(* Logix 5000 AddOnInstructionDefinition export EH_Picomag_DMA_IOL; software revision 38.00 *)

TYPE EH_CommAOI_Data :
STRUCT
   Device_Comm_Error : BOOL;
   CommSuccess : BOOL;
   CommFailed : BOOL;
   CommTimeOut : BOOL;
   StateDone : BOOL;
   NewState : BOOL;
   OldState : SINT;
   PortSize : SINT;
   DevicePort : SINT;
   MaxState : SINT;
   State : SINT;
   VendorID : INT;
   DeviceID : DINT;
   CyclicData : INT[16];
   AcyclicData : DINT[8];
   ReplayIndex : INT;
   AOI_Diagnostic : DINT;
   ConnectionStatus : DINT;
   OutputData : INT[16];
END_STRUCT
END_TYPE

ADD_ON_INSTRUCTION EH_Picomag_DMA_IOL   (* revision 1.0, vendor Endress+Hauser *)
// Picomag DMA  Rev 1 IO-Link
// Picomag DMA  Rev 2 IO-Link
VAR_IN_OUT
   DataToSend : INT[10]; {required}
   CommAOIBusy : DINT; {required}
   ActiveComPort : DINT; {required}
   DeviceAOISendRequest : DINT; {required}
   CommError : INT; {required}
   DeviceData : EH_CommAOI_Data; {required}
END_VAR
VAR_OUTPUT
   qVendor_ID : DINT; {access Read Only, visible}
   qDevice_ID : DINT; {access Read Only, visible}
END_VAR
VAR_INPUT
   iExecuteRisingEdge : BOOL; {visible}
   iSetSimulation : BOOL; {visible}
   iSetResetTotalizer : BOOL; {visible}
   iSetSimulationConductivity : REAL; {visible}
   iSetSimulationVolumeflow : REAL; {visible}
   iSetSimulationTemperature : REAL; {visible}
END_VAR
VAR_OUTPUT
   qConductivity : REAL; {visible}
   qTotalizer : REAL; {access Read Only, visible}
   qVolumeflow : REAL; {visible}
   qTemperature : REAL; {visible}
   qS_Out_1 : BOOL; {access Read Only, visible}
   qS_Out_2 : BOOL; {visible}
   qSimulationActive : BOOL; {access Read Only, visible}
   qActual_Diagnostics_Code : DINT; {access Read Only, visible}
END_VAR
VAR_IN_OUT
   qActual_Diagnostics_String : STRING; {required}
END_VAR
VAR_OUTPUT
   qLast_Diagnostics_Code : DINT; {visible}
END_VAR
VAR_IN_OUT
   qLast_Diagnostics_String : STRING; {required}
END_VAR
VAR_OUTPUT
   qAOI_Diagnostic : DINT; {access Read Only, visible}
   qCommError : INT; {access None, visible}
   qCommunicationBusy : DINT; {access Read Only, visible}
   qDeviceConnectionError : BOOL; {access Read Only, visible}
END_VAR
VAR
   Calc_DID : DINT; {access None}
   Calc_VID : DINT; {access None}
   Calc_Data : DINT; {access None}
   Calc_VID_1 : DINT; {access None}
   Calc_DID_1 : DINT; {access None}
   Calc_DID_2 : DINT; {access None}
   Cond_DINT : DINT; {access None}
   Temp_DINT : DINT; {access None}
   Calc_Cond : DINT; {access None}
   Cald_Temp : DINT; {access None}
   Calc_Temp : DINT; {access None}
   Calc_CondenStatus : DINT; {access None}
   CMD_Index : INT; {access None}
   CMD_Subindex : INT; {access None}
   CMD_Rd_Wr : BOOL; {access None}
   CMD_ByteLength : INT; {access None}
   StateMax : INT; {access None}
   CMD_RdWr_Buffer : INT[15]; {access None}
   Trigger : BOOL; {access None}
   CMD_Rd : BOOL; {access None}
   CMD_Wr : BOOL; {access None}
   SimulationDINT : DINT; {access None}
   SimulationReal : DINT; {access None}
   Calc_Out : DINT; {access None}
   Calc_Vflow : DINT; {access None}
   Calc_Tota : DINT; {access None}
   Totalizer_DINT : DINT; {access None}
   Vflow_DINT : DINT; {access None}
   xTemp : REAL; {access None}
   InputByteLength : DINT; {access None}
   iState : DINT; {access None}
   AOI_Prio : BOOL; {access None}
   ActiveAOI : BOOL; {access None}
   StateMin : INT; {access None}
   qDevice_ID_select : INT; {access None}
   DeviceID1 : DINT; {access None}
   firstTimeDone : BOOL; {access None}
   Calc_Connection_Status : DINT; {access None}
   ChangedStatus : BOOL; {access None}
   OldStatus : DINT; {access None}
   DeviceID2 : DINT; {access None}
   FALSE : BOOL; {access None}
   TRUE : BOOL := 1; {access None}
END_VAR

ROUTINE Logic   (* structured text *)
// Picomag Communication via AL1323
   // =======================================================================
   // Endress+Hauser Digital Solutions
   // ©Copyright (2024) All Rights Reserved
   // =======================================================================
   // Name:                EH_Picomag_DMA_IOL
   // Version:             1.0
   // Datum:               11.2025
   // Library:             01.01.00
   // Engineering:         Studio5000 V38.00.00
   // Author:              EH
   // =======================================================================
   
   
   qAOI_Diagnostic := DeviceData.AOI_Diagnostic;
   qCommunicationBusy := CommAOIBusy;
   DeviceID1 := 65792;  //0x94FF DevRev 2
   DeviceID2 := 65793;  //0x94FF DevRev 1
   StateMin := 0;
   DeviceData.MaxState := 9;
   
   if DeviceData.DevicePort = 0 or DeviceData.DeviceID < DeviceID1 or DeviceData.DeviceID > DeviceID2 or DeviceData.ConnectionStatus <> 1 then
   
   	qVendor_ID	:= 0;
   	qDevice_ID	:= 0;
   	qConductivity	:= 0;
   	qTotalizer	:= 0;
   	qVolumeflow	:= 0;
   	qTemperature	:= 0;
   	qS_Out_1	:= 0;
   	qS_Out_2	:= 0;
   	qSimulationActive	:= 0;
   	qActual_Diagnostics_Code	:= 0;
   	qLast_Diagnostics_Code	:= 0;
   	qLast_Diagnostics_String	:= '';
   
   	if DeviceData.DevicePort = 0 then
   
   		qActual_Diagnostics_String	:= 'Device Port is Zero';
   		DeviceData.AOI_Diagnostic.1 := TRUE;
   
   	elsif DeviceData.ConnectionStatus <> 1 then
   
   		qActual_Diagnostics_String	:= 'No Device connected';
   		qDeviceConnectionError := TRUE;
   
   	elsif DeviceData.DeviceID < DeviceID1 or DeviceData.DeviceID > DeviceID2  then
   
   		qActual_Diagnostics_String	:= 'Wrong DeviceID';
   		DeviceData.AOI_Diagnostic.2 := TRUE;
   		qVendor_ID := DeviceData.VendorID;
   		qDevice_ID := DeviceData.DeviceID;
   
   	end_if;
   
   else
   
   	if qActual_Diagnostics_Code = 0 then
   
   		qActual_Diagnostics_String	:= '--------';
   
   	end_if;
   
   	if qLast_Diagnostics_Code = 0 then
   
   		qLast_Diagnostics_String	:= '--------';
   
   	end_if;
   
   	DeviceData.AOI_Diagnostic.1 := FALSE;
   	qDeviceConnectionError := FALSE;
   	DeviceData.AOI_Diagnostic.2  := FALSE;
   
   end_if;
   
   
   if not DeviceData.AOI_Diagnostic.0
   	and not qDeviceConnectionError
   	and not DeviceData.AOI_Diagnostic.2
   	and DeviceData.DevicePort > 0 or ActiveAOI and qDeviceConnectionError then
   
   	//*********************************
   	//Vendor ID
   	//*********************************
   
   	qVendor_ID := DeviceData.VendorID;
   
   	//*********************************
   	//Device ID
   	//*********************************
   	if DeviceData.DeviceID = DeviceID1 then
   
   		qDevice_ID_select := 1;
   
   	elsif DeviceData.DeviceID = DeviceID2 then
   
   		qDevice_ID_select := 2;
   
   	else
   
   		qDevice_ID_select := 0;
   
   	end_if;
   
   	qDevice_ID := DeviceData.DeviceID;
   
   	case qDevice_ID_select of
   
   		//*********************************
   		1: // Picomag Rev 1
   		//*********************************
   
   			Calc_Tota 	:= 0+((DeviceData.DevicePort-1)*InputByteLength);  // Value  95 + Protnumber x Datalength in Byte
   			Calc_Vflow 	:= 2+((DeviceData.DevicePort-1)*InputByteLength);  // Value  97 + Protnumber x Datalength in Byte
   			Calc_Temp 	:= 4+((DeviceData.DevicePort-1)*InputByteLength);  // Value  99 + Protnumber x Datalength in Byte
   			Calc_Out 	:= 4+((DeviceData.DevicePort-1)*InputByteLength); // Value  99 + Protnumber x Datalength in Byte
   			// Temp und Out are in the Same 2 byte
   
   			//*********************************
   			//Process Data Totalizer
   			//*********************************
   
   			Totalizer_DINT		:= DeviceData.CyclicData[Calc_Tota+1];
   			Totalizer_DINT.8	:= DeviceData.CyclicData[Calc_Tota+1].8;
   			Totalizer_DINT.9 	:= DeviceData.CyclicData[Calc_Tota+1].9;
   			Totalizer_DINT.10	:= DeviceData.CyclicData[Calc_Tota+1].10;
   			Totalizer_DINT.11	:= DeviceData.CyclicData[Calc_Tota+1].11;
   			Totalizer_DINT.12 	:= DeviceData.CyclicData[Calc_Tota+1].12;
   			Totalizer_DINT.13	:= DeviceData.CyclicData[Calc_Tota+1].13;
   			Totalizer_DINT.14	:= DeviceData.CyclicData[Calc_Tota+1].14;
   			Totalizer_DINT.15	:= DeviceData.CyclicData[Calc_Tota+1].15;
   			Totalizer_DINT.16	:= DeviceData.CyclicData[Calc_Tota].0;
   			Totalizer_DINT.17	:= DeviceData.CyclicData[Calc_Tota].1;
   			Totalizer_DINT.18	:= DeviceData.CyclicData[Calc_Tota].2;
   			Totalizer_DINT.19	:= DeviceData.CyclicData[Calc_Tota].3;
   			Totalizer_DINT.20	:= DeviceData.CyclicData[Calc_Tota].4;
   			Totalizer_DINT.21	:= DeviceData.CyclicData[Calc_Tota].5;
   			Totalizer_DINT.22	:= DeviceData.CyclicData[Calc_Tota].6;
   			Totalizer_DINT.23	:= DeviceData.CyclicData[Calc_Tota].7;
   			Totalizer_DINT.24	:= DeviceData.CyclicData[Calc_Tota].8;
   			Totalizer_DINT.25	:= DeviceData.CyclicData[Calc_Tota].9;
   			Totalizer_DINT.26	:= DeviceData.CyclicData[Calc_Tota].10;
   			Totalizer_DINT.27	:= DeviceData.CyclicData[Calc_Tota].11;
   			Totalizer_DINT.28	:= DeviceData.CyclicData[Calc_Tota].12;
   			Totalizer_DINT.29	:= DeviceData.CyclicData[Calc_Tota].13;
   			Totalizer_DINT.30	:= DeviceData.CyclicData[Calc_Tota].14;
   			Totalizer_DINT.31	:= DeviceData.CyclicData[Calc_Tota].15;
   
   			COP(Totalizer_DINT,qTotalizer,1);
   
   			//*********************************
   			//Process Data Volumeflow
   			//*********************************
   
   			Vflow_DINT		:= DeviceData.CyclicData[Calc_Vflow+1];
   			Vflow_DINT.8	:= DeviceData.CyclicData[Calc_Vflow+1].8;
   			Vflow_DINT.9	:= DeviceData.CyclicData[Calc_Vflow+1].9;
   			Vflow_DINT.10	:= DeviceData.CyclicData[Calc_Vflow+1].10;
   			Vflow_DINT.11	:= DeviceData.CyclicData[Calc_Vflow+1].11;
   			Vflow_DINT.12	:= DeviceData.CyclicData[Calc_Vflow+1].12;
   			Vflow_DINT.13	:= DeviceData.CyclicData[Calc_Vflow+1].13;
   			Vflow_DINT.14	:= DeviceData.CyclicData[Calc_Vflow+1].14;
   			Vflow_DINT.15	:= DeviceData.CyclicData[Calc_Vflow+1].15;
   			Vflow_DINT.16	:= DeviceData.CyclicData[Calc_Vflow].0;
   			Vflow_DINT.17	:= DeviceData.CyclicData[Calc_Vflow].1;
   			Vflow_DINT.18	:= DeviceData.CyclicData[Calc_Vflow].2;
   			Vflow_DINT.19	:= DeviceData.CyclicData[Calc_Vflow].3;
   			Vflow_DINT.20	:= DeviceData.CyclicData[Calc_Vflow].4;
   			Vflow_DINT.21	:= DeviceData.CyclicData[Calc_Vflow].5;
   			Vflow_DINT.22	:= DeviceData.CyclicData[Calc_Vflow].6;
   			Vflow_DINT.23	:= DeviceData.CyclicData[Calc_Vflow].7;
   			Vflow_DINT.24	:= DeviceData.CyclicData[Calc_Vflow].8;
   			Vflow_DINT.25	:= DeviceData.CyclicData[Calc_Vflow].9;
   			Vflow_DINT.26	:= DeviceData.CyclicData[Calc_Vflow].10;
   			Vflow_DINT.27	:= DeviceData.CyclicData[Calc_Vflow].11;
   			Vflow_DINT.28	:= DeviceData.CyclicData[Calc_Vflow].12;
   			Vflow_DINT.29	:= DeviceData.CyclicData[Calc_Vflow].13;
   			Vflow_DINT.30	:= DeviceData.CyclicData[Calc_Vflow].14;
   			Vflow_DINT.31	:= DeviceData.CyclicData[Calc_Vflow].15;
   
   			COP(Vflow_DINT,qVolumeflow,1);
   
   			//*********************************
   			// Process Parameter Temperatur
   			//*********************************
   
   			Temp_DINT.0	:= DeviceData.CyclicData[Calc_Temp].4;
   			Temp_DINT.1	:= DeviceData.CyclicData[Calc_Temp].5;
   			Temp_DINT.2	:= DeviceData.CyclicData[Calc_Temp].6;
   			Temp_DINT.3	:= DeviceData.CyclicData[Calc_Temp].7;
   			Temp_DINT.4	:= DeviceData.CyclicData[Calc_Temp].8;
   			Temp_DINT.5	:= DeviceData.CyclicData[Calc_Temp].9;
   			Temp_DINT.6	:= DeviceData.CyclicData[Calc_Temp].10;
   			Temp_DINT.7	:= DeviceData.CyclicData[Calc_Temp].11;
   			Temp_DINT.8	:= DeviceData.CyclicData[Calc_Temp].12;
   			Temp_DINT.9	:= DeviceData.CyclicData[Calc_Temp].13;
   			Temp_DINT.10:= DeviceData.CyclicData[Calc_Temp].14;
   			Temp_DINT.11:= DeviceData.CyclicData[Calc_Temp].15;
   			Temp_DINT.12:= DeviceData.CyclicData[Calc_Temp].15;
   			Temp_DINT.13:= DeviceData.CyclicData[Calc_Temp].15;
   			Temp_DINT.14:= DeviceData.CyclicData[Calc_Temp].15;
   			Temp_DINT.15:= DeviceData.CyclicData[Calc_Temp].15;
   			Temp_DINT.16:= DeviceData.CyclicData[Calc_Temp].15;
   			Temp_DINT.17:= DeviceData.CyclicData[Calc_Temp].15;
   			Temp_DINT.18:= DeviceData.CyclicData[Calc_Temp].15;
   			Temp_DINT.19:= DeviceData.CyclicData[Calc_Temp].15;
   			Temp_DINT.20:= DeviceData.CyclicData[Calc_Temp].15;
   			Temp_DINT.21:= DeviceData.CyclicData[Calc_Temp].15;
   			Temp_DINT.22:= DeviceData.CyclicData[Calc_Temp].15;
   			Temp_DINT.23:= DeviceData.CyclicData[Calc_Temp].15;
   			Temp_DINT.24:= DeviceData.CyclicData[Calc_Temp].15;
   			Temp_DINT.25:= DeviceData.CyclicData[Calc_Temp].15;
   			Temp_DINT.26:= DeviceData.CyclicData[Calc_Temp].15;
   			Temp_DINT.27:= DeviceData.CyclicData[Calc_Temp].15;
   			Temp_DINT.28:= DeviceData.CyclicData[Calc_Temp].15;
   			Temp_DINT.29:= DeviceData.CyclicData[Calc_Temp].15;
   			Temp_DINT.30:= DeviceData.CyclicData[Calc_Temp].15;
   			Temp_DINT.31:= DeviceData.CyclicData[Calc_Temp].15;
   
   			xTemp	:= Temp_DINT;
   			qTemperature := xTemp/10;
   
   			//*********************************
   			// Process Parameter State IO1 and IO2
   			//*********************************
   
   			qS_Out_1 := DeviceData.CyclicData[Calc_Out].2;
   			qS_Out_2 := DeviceData.CyclicData[Calc_Out].3;
   
   
   
   		//*********************************
   	    2: // Picomag Rev 2
   	    //*********************************
   
   			Calc_Cond 	:= 0+((DeviceData.DevicePort-1)*InputByteLength);  // Value  (95) 0 + Protnumber x Datalength in Byte
   			Calc_Tota 	:= 2+((DeviceData.DevicePort-1)*InputByteLength);  // Value  (97) 2 + Protnumber x Datalength in Byte
   			Calc_Vflow 	:= 4+((DeviceData.DevicePort-1)*InputByteLength);  // Value  (99) 4 + Protnumber x Datalength in Byte
   			Calc_Temp 	:= 6+((DeviceData.DevicePort-1)*InputByteLength); // Value  (101) 6 + Protnumber x Datalength in Byte
   			Calc_Out 	:= 7+((DeviceData.DevicePort-1)*InputByteLength); // Value  (102) 7 + Protnumber x Datalength in Byte
   
   
   			//*********************************
   			//Process Data Conductivity
   			//*********************************
   
   			Cond_DINT	:= DeviceData.CyclicData[Calc_Cond+1];
   			Cond_DINT.8	:= DeviceData.CyclicData[Calc_Cond+1].8;
   			Cond_DINT.9	:= DeviceData.CyclicData[Calc_Cond+1].9;
   			Cond_DINT.10 := DeviceData.CyclicData[Calc_Cond+1].10;
   			Cond_DINT.11 := DeviceData.CyclicData[Calc_Cond+1].11;
   			Cond_DINT.12 := DeviceData.CyclicData[Calc_Cond+1].12;
   			Cond_DINT.13 := DeviceData.CyclicData[Calc_Cond+1].13;
   			Cond_DINT.14 := DeviceData.CyclicData[Calc_Cond+1].14;
   			Cond_DINT.15 := DeviceData.CyclicData[Calc_Cond+1].15;
   			Cond_DINT.16 := DeviceData.CyclicData[Calc_Cond].0;
   			Cond_DINT.17 := DeviceData.CyclicData[Calc_Cond].1;
   			Cond_DINT.18 := DeviceData.CyclicData[Calc_Cond].2;
   			Cond_DINT.19 := DeviceData.CyclicData[Calc_Cond].3;
   			Cond_DINT.20 := DeviceData.CyclicData[Calc_Cond].4;
   			Cond_DINT.21 := DeviceData.CyclicData[Calc_Cond].5;
   			Cond_DINT.22 := DeviceData.CyclicData[Calc_Cond].6;
   			Cond_DINT.23 := DeviceData.CyclicData[Calc_Cond].7;
   			Cond_DINT.24 := DeviceData.CyclicData[Calc_Cond].8;
   			Cond_DINT.25 := DeviceData.CyclicData[Calc_Cond].9;
   			Cond_DINT.26 := DeviceData.CyclicData[Calc_Cond].10;
   			Cond_DINT.27 := DeviceData.CyclicData[Calc_Cond].11;
   			Cond_DINT.28 := DeviceData.CyclicData[Calc_Cond].12;
   			Cond_DINT.29 := DeviceData.CyclicData[Calc_Cond].13;
   			Cond_DINT.30 := DeviceData.CyclicData[Calc_Cond].14;
   			Cond_DINT.31 := DeviceData.CyclicData[Calc_Cond].15;
   
   			COP(Cond_DINT,qConductivity,1);
   
   			//*********************************
   			//Process Data Totalizer
   			//*********************************
   
   			Totalizer_DINT := DeviceData.CyclicData[Calc_Tota+1];
   			Totalizer_DINT.8 := DeviceData.CyclicData[Calc_Tota+1].8;
   			Totalizer_DINT.9 := DeviceData.CyclicData[Calc_Tota+1].9;
   			Totalizer_DINT.10 := DeviceData.CyclicData[Calc_Tota+1].10;
   			Totalizer_DINT.11 := DeviceData.CyclicData[Calc_Tota+1].11;
   			Totalizer_DINT.12 := DeviceData.CyclicData[Calc_Tota+1].12;
   			Totalizer_DINT.13 := DeviceData.CyclicData[Calc_Tota+1].13;
   			Totalizer_DINT.14 := DeviceData.CyclicData[Calc_Tota+1].14;
   			Totalizer_DINT.15 := DeviceData.CyclicData[Calc_Tota+1].15;
   			Totalizer_DINT.16 := DeviceData.CyclicData[Calc_Tota].0;
   			Totalizer_DINT.17 := DeviceData.CyclicData[Calc_Tota].1;
   			Totalizer_DINT.18 := DeviceData.CyclicData[Calc_Tota].2;
   			Totalizer_DINT.19 := DeviceData.CyclicData[Calc_Tota].3;
   			Totalizer_DINT.20 := DeviceData.CyclicData[Calc_Tota].4;
   			Totalizer_DINT.21 := DeviceData.CyclicData[Calc_Tota].5;
   			Totalizer_DINT.22 := DeviceData.CyclicData[Calc_Tota].6;
   			Totalizer_DINT.23 := DeviceData.CyclicData[Calc_Tota].7;
   			Totalizer_DINT.24 := DeviceData.CyclicData[Calc_Tota].8;
   			Totalizer_DINT.25 := DeviceData.CyclicData[Calc_Tota].9;
   			Totalizer_DINT.26 := DeviceData.CyclicData[Calc_Tota].10;
   			Totalizer_DINT.27 := DeviceData.CyclicData[Calc_Tota].11;
   			Totalizer_DINT.28 := DeviceData.CyclicData[Calc_Tota].12;
   			Totalizer_DINT.29 := DeviceData.CyclicData[Calc_Tota].13;
   			Totalizer_DINT.30 := DeviceData.CyclicData[Calc_Tota].14;
   			Totalizer_DINT.31 := DeviceData.CyclicData[Calc_Tota].15;
   
   			COP(Totalizer_DINT,qTotalizer,1);
   
   			//*********************************
   			//Process Data Volumeflow
   			//*********************************
   
   			Vflow_DINT	:= DeviceData.CyclicData[Calc_Vflow+1];
   			Vflow_DINT.8 := DeviceData.CyclicData[Calc_Vflow+1].8;
   			Vflow_DINT.9 := DeviceData.CyclicData[Calc_Vflow+1].9;
   			Vflow_DINT.10 := DeviceData.CyclicData[Calc_Vflow+1].10;
   			Vflow_DINT.11 := DeviceData.CyclicData[Calc_Vflow+1].11;
   			Vflow_DINT.12 := DeviceData.CyclicData[Calc_Vflow+1].12;
   			Vflow_DINT.13 := DeviceData.CyclicData[Calc_Vflow+1].13;
   			Vflow_DINT.14 := DeviceData.CyclicData[Calc_Vflow+1].14;
   			Vflow_DINT.15 := DeviceData.CyclicData[Calc_Vflow+1].15;
   			Vflow_DINT.16 := DeviceData.CyclicData[Calc_Vflow].0;
   			Vflow_DINT.17 := DeviceData.CyclicData[Calc_Vflow].1;
   			Vflow_DINT.18 := DeviceData.CyclicData[Calc_Vflow].2;
   			Vflow_DINT.19 := DeviceData.CyclicData[Calc_Vflow].3;
   			Vflow_DINT.20 := DeviceData.CyclicData[Calc_Vflow].4;
   			Vflow_DINT.21 := DeviceData.CyclicData[Calc_Vflow].5;
   			Vflow_DINT.22 := DeviceData.CyclicData[Calc_Vflow].6;
   			Vflow_DINT.23 := DeviceData.CyclicData[Calc_Vflow].7;
   			Vflow_DINT.24 := DeviceData.CyclicData[Calc_Vflow].8;
   			Vflow_DINT.25 := DeviceData.CyclicData[Calc_Vflow].9;
   			Vflow_DINT.26 := DeviceData.CyclicData[Calc_Vflow].10;
   			Vflow_DINT.27 := DeviceData.CyclicData[Calc_Vflow].11;
   			Vflow_DINT.28 := DeviceData.CyclicData[Calc_Vflow].12;
   			Vflow_DINT.29 := DeviceData.CyclicData[Calc_Vflow].13;
   			Vflow_DINT.30 := DeviceData.CyclicData[Calc_Vflow].14;
   			Vflow_DINT.31 := DeviceData.CyclicData[Calc_Vflow].15;
   
   			COP(Vflow_DINT,qVolumeflow,1);
   
   			//*********************************
   			// Process Parameter Temperatur
   			//*********************************
   
   			Temp_DINT	:= DeviceData.CyclicData[Calc_Temp];
   			xTemp		:= Temp_DINT;
   			qTemperature:= xTemp/10;
   
   
   			//*********************************
   			// Process Parameter State IO1 and IO2
   			//*********************************
   
   			qS_Out_1 := DeviceData.CyclicData[Calc_Out].10;
   			qS_Out_2 := DeviceData.CyclicData[Calc_Out].11;
   
   		end_case;
   
   
   	//*********************************
   	// Checking for CommBlockBusy
   	//*********************************
   
   
   	if iExecuteRisingEdge and DeviceData.State = 0 then
   
   		DeviceAOISendRequest.[DeviceData.DevicePort] := 1;
   
   	end_if;
   
   
   	if ActiveComPort = DeviceData.DevicePort then
   
   		AOI_Prio :=1;
   	else
   
   		AOI_Prio := 0;
   	end_if;
   
   
   	if CommAOIBusy = 1 and iExecuteRisingEdge and DeviceData.State = 0 and AOI_Prio then
   
   		ActiveAOI := 1;
   
   
   	end_if;
   
   
   	qCommunicationBusy := CommAOIBusy;
   	qAOI_Diagnostic := DeviceData.AOI_Diagnostic;
   
   	if  ActiveAOI and qDeviceConnectionError then
   
   		DeviceData.State := DeviceData.MaxState;
   
   	end_if;
   
   	//*********************************
   	// State machine
   	//*********************************
   
   	if ActiveAOI or DeviceData.State = DeviceData.MaxState then
   
   	case DeviceData.State of
   
   		//*********************************
   	    0: // Idle
   	    //*********************************
   
   		    // Initializing reset to O for CMD Relevant Settings
   		    Trigger := 0;
   			CMD_Index := 0;
   			CMD_Subindex := 0;
   			CMD_Wr := 0;
   			CMD_Rd := 0;
   		    CMD_ByteLength := 0;
   
   			IF DeviceData.DevicePort = ActiveComPort then // check if Device is Active to reset success
   					DeviceData.CommSuccess := 0;
   					DeviceData.CommTimeOut := 0;
   					DeviceData.NewState := 1;
   					DeviceData.StateDone := 0;
   			end_if;
   
   		    // Wait for trigger
   		    if iExecuteRisingEdge and ActiveComPort = DeviceData.DevicePort then
   
   				DeviceData.AOI_Diagnostic := 0;
   				DeviceData.State := DeviceData.State + 1;
   
   		    end_if;
   
   	    //*********************************
   	    1: // Simulation
   	    //*********************************
   
   		    CMD_Index := 351;
   		    CMD_Subindex := 0;
   		    CMD_Wr := 1;
   			CMD_Rd := 0;
   		    CMD_ByteLength := 2;
   			DataToSend[6]:= 0;
   			DataToSend[7]:= 0;
   
   		    if iSetSimulation then
   
   			   DataToSend[6].8 := 1;
   
   			else
   
   			    DataToSend[6].8 := 0;
   
   			end_if;
   
   		    Trigger := 1;
   
   			if DeviceData.NewState then
   
   				DeviceData.StateDone := 1;
   
   			end_if;
   
   			if  DeviceData.CommSuccess and DeviceData.ReplayIndex = CMD_Index then
   
   				Trigger := 0;
   		        DeviceData.State := DeviceData.State + 1;
   				DeviceData.CommSuccess := 0;
   				DeviceData.AcyclicData[0] := 0;
   				DeviceData.NewState := 1;
   
   			 elsif DeviceData.CommTimeOut then
   
   				DeviceData.AOI_Diagnostic.[DeviceData.State+7] := 1;
   				Trigger := 0;
   		        DeviceData.State := DeviceData.State + 1;
   				DeviceData.CommTimeOut := 0;
   				DeviceData.AcyclicData[0] := 0;
   				DeviceData.NewState := 1;
   
   		    end_if;
   
   	    //*********************************
   	    2: // Simulation - Value VolumeFlow
   	    //*********************************
   
   		    CMD_Index := 358;
   		    CMD_Subindex := 0;
   		    CMD_Wr := 1;
   			CMD_Rd := 0;
   		    CMD_ByteLength := 4;
   
   			COP(iSetSimulationVolumeflow,SimulationDINT,1); // Copy the Bits of the REAL in a DINT not the Value
   
   			DataToSend[6].0 :=  SimulationDINT.24;
   			DataToSend[6].1 :=  SimulationDINT.25;
   			DataToSend[6].2 :=  SimulationDINT.26;
   			DataToSend[6].3 :=  SimulationDINT.27;
   			DataToSend[6].4 :=  SimulationDINT.28;
   			DataToSend[6].5 :=  SimulationDINT.29;
   			DataToSend[6].6 :=  SimulationDINT.30;
   			DataToSend[6].7 :=  SimulationDINT.31;
   			DataToSend[6].8 :=  SimulationDINT.16;
   			DataToSend[6].9 :=  SimulationDINT.17;
   			DataToSend[6].10 := SimulationDINT.18;
   			DataToSend[6].11 := SimulationDINT.19;
   			DataToSend[6].12 := SimulationDINT.20;
   			DataToSend[6].13 := SimulationDINT.21;
   			DataToSend[6].14 := SimulationDINT.22;
   			DataToSend[6].15 := SimulationDINT.23;
   			DataToSend[7].0  := SimulationDINT.8;
   			DataToSend[7].1  := SimulationDINT.9;
   			DataToSend[7].2  := SimulationDINT.10;
   			DataToSend[7].3  := SimulationDINT.11;
   			DataToSend[7].4  := SimulationDINT.12;
   			DataToSend[7].5  := SimulationDINT.13;
   			DataToSend[7].6  := SimulationDINT.14;
   			DataToSend[7].7  := SimulationDINT.15;
   			DataToSend[7].8  := SimulationDINT.0;
   			DataToSend[7].9  := SimulationDINT.1;
   			DataToSend[7].10 := SimulationDINT.2;
   			DataToSend[7].11 := SimulationDINT.3;
   			DataToSend[7].12 := SimulationDINT.4;
   			DataToSend[7].13 := SimulationDINT.5;
   			DataToSend[7].14 := SimulationDINT.6;
   			DataToSend[7].15 := SimulationDINT.7;
   
   		    Trigger := 1;
   
   			if DeviceData.NewState then
   
   				DeviceData.StateDone := 1;
   
   			end_if;
   
   			if  DeviceData.CommSuccess and DeviceData.ReplayIndex = CMD_Index then
   
   				Trigger := 0;
   		        DeviceData.State := DeviceData.State + 1;
   				DeviceData.CommSuccess := 0;
   				DeviceData.AcyclicData[0] := 0;
   				DeviceData.NewState := 1;
   
   			elsif DeviceData.CommTimeOut then
   
   				DeviceData.AOI_Diagnostic.[DeviceData.State+7] := 1;
   				Trigger := 0;
   		        DeviceData.State := DeviceData.State + 1;
   				DeviceData.CommTimeOut := 0;
   				DeviceData.AcyclicData[0] := 0;
   				DeviceData.NewState := 1;
   
   		    end_if;
   
   
   		//*********************************
   	    3: // Simulation - Value Temperature
   	    //*********************************
   
   		    CMD_Index := 360;
   		    CMD_Subindex := 0;
   		    CMD_Wr := 1;
   			CMD_Rd := 0;
   		    CMD_ByteLength := 4;
   
   			COP(iSetSimulationTemperature,SimulationDINT,1); // Copy the Bits of the REAL in a DINT not the Value
   
   			DataToSend[6].0 :=  SimulationDINT.24;
   			DataToSend[6].1 :=  SimulationDINT.25;
   			DataToSend[6].2 :=  SimulationDINT.26;
   			DataToSend[6].3 :=  SimulationDINT.27;
   			DataToSend[6].4 :=  SimulationDINT.28;
   			DataToSend[6].5 :=  SimulationDINT.29;
   			DataToSend[6].6 :=  SimulationDINT.30;
   			DataToSend[6].7 :=  SimulationDINT.31;
   			DataToSend[6].8 :=  SimulationDINT.16;
   			DataToSend[6].9 :=  SimulationDINT.17;
   			DataToSend[6].10 := SimulationDINT.18;
   			DataToSend[6].11 := SimulationDINT.19;
   			DataToSend[6].12 := SimulationDINT.20;
   			DataToSend[6].13 := SimulationDINT.21;
   			DataToSend[6].14 := SimulationDINT.22;
   			DataToSend[6].15 := SimulationDINT.23;
   			DataToSend[7].0  := SimulationDINT.8;
   			DataToSend[7].1  := SimulationDINT.9;
   			DataToSend[7].2  := SimulationDINT.10;
   			DataToSend[7].3  := SimulationDINT.11;
   			DataToSend[7].4  := SimulationDINT.12;
   			DataToSend[7].5  := SimulationDINT.13;
   			DataToSend[7].6  := SimulationDINT.14;
   			DataToSend[7].7  := SimulationDINT.15;
   			DataToSend[7].8  := SimulationDINT.0;
   			DataToSend[7].9  := SimulationDINT.1;
   			DataToSend[7].10 := SimulationDINT.2;
   			DataToSend[7].11 := SimulationDINT.3;
   			DataToSend[7].12 := SimulationDINT.4;
   			DataToSend[7].13 := SimulationDINT.5;
   			DataToSend[7].14 := SimulationDINT.6;
   			DataToSend[7].15 := SimulationDINT.7;
   
   		    Trigger := 1;
   
   			if DeviceData.NewState then
   
   				DeviceData.StateDone := 1;
   
   			end_if;
   
   			if  DeviceData.CommSuccess and DeviceData.ReplayIndex = CMD_Index then
   
   				Trigger := 0;
   		        DeviceData.State := DeviceData.State + 1;
   				DeviceData.CommSuccess := 0;
   				DeviceData.AcyclicData[0] := 0;
   				DeviceData.NewState := 1;
   
   			elsif DeviceData.CommTimeOut then
   
   				DeviceData.AOI_Diagnostic.[DeviceData.State+7] := 1;
   				Trigger := 0;
   		        DeviceData.State := DeviceData.State + 1;
   				DeviceData.CommTimeOut := 0;
   				DeviceData.AcyclicData[0] := 0;
   				DeviceData.NewState := 1;
   
   		    end_if;
   
   		//*********************************
   	    4: // Simulation - Value Conductivity
   	    //*********************************
   
   		    CMD_Index := 359;
   		    CMD_Subindex := 0;
   		    CMD_Wr := 1;
   			CMD_Rd := 0;
   		    CMD_ByteLength := 4;
   
   			COP(iSetSimulationConductivity,SimulationDINT,1); // Copie the Bits from the Real in a DINT
   
   			DataToSend[6].0 :=  SimulationDINT.24;
   			DataToSend[6].1 :=  SimulationDINT.25;
   			DataToSend[6].2 :=  SimulationDINT.26;
   			DataToSend[6].3 :=  SimulationDINT.27;
   			DataToSend[6].4 :=  SimulationDINT.28;
   			DataToSend[6].5 :=  SimulationDINT.29;
   			DataToSend[6].6 :=  SimulationDINT.30;
   			DataToSend[6].7 :=  SimulationDINT.31;
   			DataToSend[6].8 :=  SimulationDINT.16;
   			DataToSend[6].9 :=  SimulationDINT.17;
   			DataToSend[6].10 := SimulationDINT.18;
   			DataToSend[6].11 := SimulationDINT.19;
   			DataToSend[6].12 := SimulationDINT.20;
   			DataToSend[6].13 := SimulationDINT.21;
   			DataToSend[6].14 := SimulationDINT.22;
   			DataToSend[6].15 := SimulationDINT.23;
   			DataToSend[7].0  := SimulationDINT.8;
   			DataToSend[7].1  := SimulationDINT.9;
   			DataToSend[7].2  := SimulationDINT.10;
   			DataToSend[7].3  := SimulationDINT.11;
   			DataToSend[7].4  := SimulationDINT.12;
   			DataToSend[7].5  := SimulationDINT.13;
   			DataToSend[7].6  := SimulationDINT.14;
   			DataToSend[7].7  := SimulationDINT.15;
   			DataToSend[7].8  := SimulationDINT.0;
   			DataToSend[7].9  := SimulationDINT.1;
   			DataToSend[7].10 := SimulationDINT.2;
   			DataToSend[7].11 := SimulationDINT.3;
   			DataToSend[7].12 := SimulationDINT.4;
   			DataToSend[7].13 := SimulationDINT.5;
   			DataToSend[7].14 := SimulationDINT.6;
   			DataToSend[7].15 := SimulationDINT.7;
   
   		    Trigger := 1;
   
   			if DeviceData.NewState then
   
   				DeviceData.StateDone := 1;
   
   			end_if;
   
   			if  DeviceData.CommSuccess and DeviceData.ReplayIndex = CMD_Index then
   
   				Trigger := 0;
   		        DeviceData.State := DeviceData.State + 1;
   				DeviceData.CommSuccess := 0;
   				DeviceData.AcyclicData[0] := 0;
   				DeviceData.NewState := 1;
   
   			elsif DeviceData.CommTimeOut then
   
   				DeviceData.AOI_Diagnostic.[DeviceData.State+7] := 1;
   				Trigger := 0;
   		        DeviceData.State := DeviceData.State + 1;
   				DeviceData.CommTimeOut := 0;
   				DeviceData.AcyclicData[0] := 0;
   				DeviceData.NewState := 1;
   
   		    end_if;
   
   		//*********************************
   	    5: // Reset Totalizer
   	    //*********************************
   
   		    CMD_Index := 362;
   		    CMD_Subindex := 0;
   		    CMD_Wr := 1;
   			CMD_Rd := 0;
   		    CMD_ByteLength := 2;
   			DataToSend[6] := 0;
   			DataToSend[7]:= 0;
   
   			If iSetResetTotalizer then
   
   			    DataToSend[6].8 := 1;
   
   			end_if;
   
   		    Trigger := 1;
   
   			if DeviceData.NewState then
   
   				DeviceData.StateDone := 1;
   
   			end_if;
   
   			if  DeviceData.CommSuccess and DeviceData.ReplayIndex = CMD_Index then
   
   				Trigger := 0;
   		        DeviceData.State := DeviceData.State + 1;
   				DeviceData.CommSuccess := 0;
   				DeviceData.AcyclicData[0] := 0;
   				DeviceData.NewState := 1;
   
   
   			elsif DeviceData.CommTimeOut then
   
   				DeviceData.AOI_Diagnostic.[DeviceData.State+7] := 1;
   				Trigger := 0;
   		        DeviceData.State := DeviceData.State + 1;
   				DeviceData.CommTimeOut := 0;
   				DeviceData.AcyclicData[0] := 0;
   				DeviceData.NewState := 1;
   
   		    end_if;
   
   		//*********************************
   	    6: // Simulation - SimulationActive
   	    //*********************************
   
   		    CMD_Index := 351;
   		    CMD_Subindex := 0;
   		    CMD_Wr := 0;
   			CMD_Rd := 1;
   		    CMD_ByteLength := 1;
   		    Trigger := 1;
   
   			if DeviceData.NewState then
   
   				DeviceData.StateDone := 1;
   
   			end_if;
   
   			if  DeviceData.CommSuccess and DeviceData.ReplayIndex = CMD_Index then
   
   				qSimulationActive := DeviceData.AcyclicData[0].0;
   				Trigger := 0;
   		        DeviceData.State := DeviceData.State + 1;
   				DeviceData.CommSuccess := 0;
   				DeviceData.AcyclicData[0] := 0;
   				DeviceData.NewState := 1;
   
   			elsif DeviceData.CommTimeOut then
   
   				DeviceData.AOI_Diagnostic.[DeviceData.State+7] := 1;
   				Trigger := 0;
   		        DeviceData.State := DeviceData.State + 1;
   				DeviceData.CommTimeOut := 0;
   				DeviceData.AcyclicData[0] := 0;
   				DeviceData.NewState := 1;
   
   		    end_if;
   
   		//*********************************
   		7: // Actual Diagnostic
   		//*********************************
   
   		    CMD_Index := 260;
   		    CMD_Subindex := 0;
   		    CMD_Wr := 0;
   			CMD_Rd := 1;
   			CMD_ByteLength := 2;
   		    Trigger := 1;
   
   			if DeviceData.NewState then
   
   				DeviceData.StateDone := 1;
   
   			end_if;
   
   			if  DeviceData.CommSuccess and DeviceData.ReplayIndex = CMD_Index then
   
   				qActual_Diagnostics_Code	:= DeviceData.AcyclicData[0];
   
   
   				case qActual_Diagnostics_Code of
   
   				    16#0000_0000:
   						qActual_Diagnostics_String := 'SYSTEM OK';
   					16#0000_0001:
   						qActual_Diagnostics_String := 'no communication';
   					16#4631_3831:
   						qActual_Diagnostics_String := 'F181 COIL CIRC.FAIL.';
   					16#4631_3830:
   						qActual_Diagnostics_String := 'F180 TEMP.CIRC.FAIL';
   					16#4632_3031:
   						qActual_Diagnostics_String := 'F201 DEVICE FAIL.';
   					16#4632_3033:
   						qActual_Diagnostics_String := 'F283 MEMORY FAIL.';
   					16#4334_3436:
   						qActual_Diagnostics_String := 'C446 I/O 1 OVERLOAD';
   					16#4334_3437:
   						qActual_Diagnostics_String := 'C447 I/O 2 OVERLOAD';
   					16#4334_3835:
   						qActual_Diagnostics_String := 'C485 SIMULATION ACT.';
   					16#4334_3533:
   						qActual_Diagnostics_String := 'C453 FLOW OVERRIDE';
   					16#5334_3431:
   						qActual_Diagnostics_String := 'S441 I-OUT 1 RANGE';
   					16#5334_3434:
   						qActual_Diagnostics_String := 'S444 U-OUT 1 RANGE';
   					16#5334_3433:
   						qActual_Diagnostics_String := 'S443 P-OUT 1 RANGE';
   					16#5334_3432:
   						qActual_Diagnostics_String := 'S442 I-OUT 2 RANGE';
   					16#5334_3435:
   						qActual_Diagnostics_String := 'S445 U-OUT 2 RANGE';
   					16#5339_3632:
   						qActual_Diagnostics_String := 'S962 EMPTY PIPE';
   					16#5338_3334:
   						qActual_Diagnostics_String := 'S834 TEMPERAT. RANGE ';
   					else
   						qActual_Diagnostics_String := 'Error Code unknown';
   
   				end_case;
   
   
   				Trigger := 0;
   		        DeviceData.State := DeviceData.State + 1;
   				DeviceData.CommSuccess := 0;
   				DeviceData.AcyclicData[0] := 0;
   				DeviceData.NewState := 1;
   
   			elsif DeviceData.CommTimeOut then
   
   				DeviceData.AOI_Diagnostic.[DeviceData.State+7] := 1;
   				Trigger := 0;
   		        DeviceData.State := DeviceData.State + 1;
   				DeviceData.CommTimeOut := 0;
   				DeviceData.AcyclicData[0] := 0;
   				DeviceData.NewState := 1;
   
   		    end_if;
   
   		//*********************************
   	    8: // Last Diagnostic
   	    //*********************************
   
   		    CMD_Index := 261;
   			CMD_Subindex := 0;
   		    CMD_Wr := 0;
   			CMD_Rd := 1;
   			CMD_ByteLength := 2;
   		    Trigger := 1;
   
   			if DeviceData.NewState then
   
   				DeviceData.StateDone := 1;
   
   			end_if;
   
   			if  DeviceData.CommSuccess and DeviceData.ReplayIndex = CMD_Index then
   
   				qLast_Diagnostics_Code := DeviceData.AcyclicData[0];
   
   				case qLast_Diagnostics_Code of
   
   					16#0000_0000:
   						qLast_Diagnostics_String := 'SYSTEM OK';
   					16#0000_0001:
   						qLast_Diagnostics_String := 'no communication';
   					16#4631_3831:
   						qLast_Diagnostics_String := 'F181 COIL CIRC.FAIL.';
   					16#4631_3830:
   						qLast_Diagnostics_String := 'F180 TEMP.CIRC.FAIL';
   					16#4632_3031:
   						qLast_Diagnostics_String := 'F201 DEVICE FAIL.';
   					16#4632_3033:
   						qLast_Diagnostics_String := 'F283 MEMORY FAIL.';
   					16#4334_3436:
   						qLast_Diagnostics_String := 'C446 I/O 1 OVERLOAD';
   					16#4334_3437:
   						qLast_Diagnostics_String := 'C447 I/O 2 OVERLOAD';
   					16#4334_3835:
   						qLast_Diagnostics_String := 'C485 SIMULATION ACT.';
   					16#4334_3533:
   						qLast_Diagnostics_String := 'C453 FLOW OVERRIDE';
   					16#5334_3431:
   						qLast_Diagnostics_String := 'S441 I-OUT 1 RANGE';
   					16#5334_3434:
   						qLast_Diagnostics_String := 'S444 U-OUT 1 RANGE';
   					16#5334_3433:
   						qLast_Diagnostics_String := 'S443 P-OUT 1 RANGE';
   					16#5334_3432:
   						qLast_Diagnostics_String := 'S442 I-OUT 2 RANGE';
   					16#5334_3435:
   						qLast_Diagnostics_String := 'S445 U-OUT 2 RANGE';
   					16#5339_3632:
   						qLast_Diagnostics_String := 'S962 EMPTY PIPE';
   					16#5338_3334:
   						qLast_Diagnostics_String := 'S834 TEMPERAT. RANGE ';
   					else
   						qLast_Diagnostics_String := 'Error Code unknown';
   
   				end_case;
   
   
   				Trigger := 0;
   		        DeviceData.State := DeviceData.State + 1;
   				DeviceData.CommSuccess := 0;
   				DeviceData.AcyclicData[0] := 0;
   				DeviceData.NewState := 1;
   
   			elsif DeviceData.CommTimeOut then
   
   				DeviceData.AOI_Diagnostic.[DeviceData.State+7] := 1;
   				Trigger := 0;
   		        DeviceData.State := DeviceData.State + 1;
   				DeviceData.CommTimeOut := 0;
   				DeviceData.AcyclicData[0] := 0;
   				DeviceData.NewState := 1;
   
   		    end_if;
   
   		//*********************************
   	    9: //  Trigger guard
   	    //*********************************
   
   			if not firstTimeDone then
   
   				CommAOIBusy := 0;
   				firstTimeDone := 1;
   				DeviceAOISendRequest.[DeviceData.DevicePort] := 0;
   				ActiveComPort := 0;
   				ActiveAOI := 0;
   				DataToSend[0] := 0;
   				DataToSend[1] := 0;
   				DataToSend[2] := 0;
   				DataToSend[3] := 0;
   				DataToSend[4] := 0;
   				DataToSend[5] := 0;
   				DataToSend[6] := 0;
   				DataToSend[7] := 0;
   				DataToSend[8] := 0;
   				DataToSend[9] := 0;
   				DeviceData.StateDone := 0;
   
   			end_if;
   
   			if DeviceData.State = DeviceData.MaxState AND NOT iExecuteRisingEdge then
   
   				DeviceData.State := 0;
   				DeviceData.OldState := DeviceData.State;
   				firstTimeDone := 0;
   
   			end_if;
   
   	end_case;
   
   	end_if;
   
   
   	//*************************
   	// Write Commands to the Master and the Device
   	//*************************
   	if DeviceData.State > StateMin and DeviceData.State < DeviceData.MaxState then
   
   
   	DataToSend[2] := DeviceData.DevicePort;
   	DataToSend[3] := CMD_Index;
   	DataToSend[4] := CMD_Subindex;
   	DataToSend[5].0 := CMD_Rd;
   	DataToSend[5].1 := CMD_Wr;
   	DataToSend[5].8 := CMD_ByteLength.0;  // Bits for the Length of the Data
   	DataToSend[5].9 := CMD_ByteLength.1;
   	DataToSend[5].10 := CMD_ByteLength.2;
   	DataToSend[5].11 := CMD_ByteLength.3;
   	DataToSend[5].12 := CMD_ByteLength.4;
   	DataToSend[5].13 := CMD_ByteLength.5;
   	DataToSend[5].14 := CMD_ByteLength.6;
   	DataToSend[5].15 := CMD_ByteLength.7;
   
   	DataToSend[5].7 := Trigger;
   
   
   	qCommError	:= CommError;
   
   	end_if;
   
   
   
   end_if;
END_ROUTINE
END_ADD_ON_INSTRUCTION
